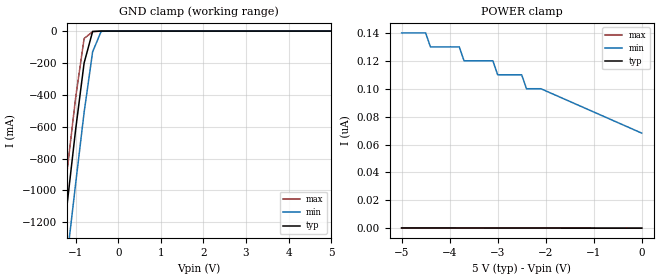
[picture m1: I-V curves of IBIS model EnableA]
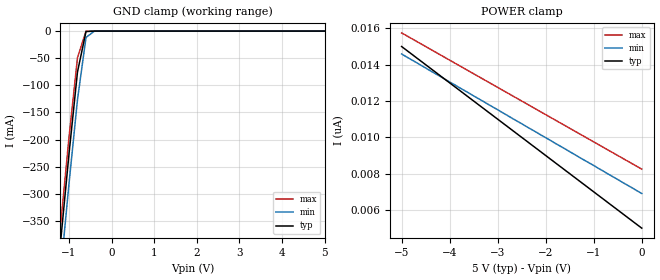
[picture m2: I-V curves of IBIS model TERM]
| I/O Buffer Information Specification (IBIS) Version 3.2 (August 20, 1999)
| IBIS is a standard for electronic behavioral specifications of integrated
| circuit input/output analog characteristics.
[IBIS Ver]   3.2
[File name]   qs3244.ibs
[File Rev]   2.0
[Date]   December 5, 2003
[Source]   From QSI silicon model
[Notes]   1. Temperatures: typ=25C, min=-40C, max=100C
   2. QSI's 0.8um SPDM process
   3. I/O model type changed to Series_switch for Data I/Os
[Disclaimer]
Integrated Device Technology, Inc. ("IDT") hereby grants the user of this
IBIS model ("User") a non-exclusive, nontransferable license to use this
IBIS model under the following terms: The User is granted this license only
to use the IBIS model for demonstration purposes only and is not granted
rights to sell, copy (except as needed to run the IBIS model), rent, lease
or sub-license (except for demonstration) the IBIS model in whole or in
part, or in modified form to anyone. The User may modify the IBIS model to
suit its specific applications, but  rights to derivative works and such
modifications shall belong to IDT.
THIS IBIS MODEL IS PROVIDED ON AN AS IS" BASIS AND IDT  MAKES ABSOLUTELY NO
WARRANTY WITH RESPECT TO THE INFORMATION CONTAINED HEREIN.  IDT DISCLAIMS
AND USER WAIVES ALL WARRANTIES, EXPRESS AND IMPLIED, INCLUDING WARRANTIES OF
MERCHANTABILITY AND FITNESS FOR A PARTICULAR PURPOSE.  THE ENTIRE RISK AS TO
QUALITY AND PERFORMANCE IS WITH THE USER  ACCORDINGLY, IN NO EVENT SHALL IDT
BE LIABLE FOR ANY DIRECT OR INDIRECT DAMAGES, WHETHER IN CONTRACT OR TORT,
INCLUDING ANY LOST PROFITS OR OTHER INCIDENTAL, CONSEQUENTIAL, EXEMPLARY, OR
PUNITIVE DAMAGES ARISING OUT OF THE USE OR APPLICATION OF THE  IBIS MODEL,
WHETHER OR NOT IDT HAD NOTICE OF SUCH DAMAGES.
IDT reserves the right to make changes without notice to any product herein
to improve reliability, function, or design. IDT does not convey any license
under patent rights or any other intellectual property rights, including
those of third parties. IDT is not obligated to provide maintenance or
support for the licensed IBIS model.
This model is for High Speed CMOS Quickswitch 8-Bit Bus Switch
[Copyright]
Copyright 2002, Integrated Device Technology, Inc. All rights reserved.
|   Component qs3244
[Component]   qs3244
[Manufacturer]   Quality Semiconductor Incorporated
[Package]
| Note that R_pkg is not given
| variable   typ   min   max
| Package parasitics.  Uncomment one set.
| PDIP
R_pkg   0.00   0.00   0.00
L_pkg   8.00nH   NA   NA
C_pkg   1.20pF   NA   NA
| SOIC
|R_pkg   0.00   0.00   0.00
|L_pkg   4.00nH   NA   NA
|C_pkg   0.70pF   NA   NA
| QSOP
|R_pkg   0.00   0.00   0.00
|L_pkg   2.50nH   NA   NA
|C_pkg   0.40pF   NA   NA
[Pin]  signal_name   model_name   R_pin   L_pin   C_pin
|1   ~1G   EnableA
2   1A1   TERM
3   2Y4   TERM
4   1A2   TERM
5   2Y3   TERM
6   1A3   TERM
7   2Y2   TERM
8   1A4   TERM
9   2Y1   TERM
11   2A1   TERM
12   1Y4   TERM
13   2A2   TERM
14   1Y3   TERM
15   2A3   TERM
16   1Y2   TERM
17   2A4   TERM
18   1Y1   TERM
|19   ~2G   EnableA
10   GND   GND
20   Vcc   POWER
[Series Switch Groups]
|Function Group States
On A /
On B /
On A B /
Off A B /
[Series Pin Mapping]   pin_2   model_name   function_table_group
2   18   QSW   A
4   16   QSW   A
6   14   QSW   A
8   12   QSW   A
11   9   QSW   B
13   7   QSW   B
15   5   QSW   B
17   3   QSW   B
|   Model QSW
[Model]   QSW
Model_type   Series_switch
C_comp   5.0pF   5.0pF   5.0pF
[Temperature Range]   25.00   100.00   -40.00
[Voltage Range]   5.00V   4.75V   5.25V
[On]
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[Off]
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| Models and submodels in the file (3): EnableA (Input), TERM (Terminator), QSW (Series_switch)
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|   Model EnableA
[Model]   EnableA
Model_type   Input
Vinl =   0.80V
Vinh =   2.00V
C_comp   5.00pF   5.00pF   5.00pF
[Temperature Range]   25.00   0.12k   -40.00
[Voltage Range]   5.00V   4.50V   5.50V
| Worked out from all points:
|   GND clamp passes 1 mA (typ) near -0.49 V on its own axis
[GND_clamp]
| voltage   I(typ)   I(min)   I(max)
-5V       -10.46A    -10.75A    -10.37A
-1.4V     -1.56A     -1.9A      -1.36A
-1.2V     -1.09A     -1.42A     -880mA
-1V       -620mA     -960mA     -420mA
-800mV    -200mA     -510mA     -46.44mA
-600mV    -2.14mA    -130mA     -4.03mA
-400mV    -3.69uA    -1.72mA    -40.62uA
5V        120pA      75.77nA    120pA
[POWER_clamp]
| voltage   I(typ)   I(min)   I(max)
-5V       280pA      140nA      290pA
-4.5V     270pA      140nA      280pA
-4.4V     260pA      130nA      270pA
-3.8V     240pA      130nA      250pA
-3.7V     240pA      120nA      250pA
-3.1V     220pA      120nA      230pA
-3V       220pA      110nA      230pA
-2.5V     200pA      110nA      210pA
-2.4V     200pA      100nA      210pA
-2.1V     190pA      100nA      200pA
0V        120pA      68.19nA    130pA
|   Model TERM
[Model]   TERM
Model_type   Terminator
Polarity   Non-Inverting
C_comp   5.00pF   5.00pF   5.00pF
[Temperature Range]   25.00   100.00   -40.00
[Voltage Range]   5.0V   4.75V   5.25V
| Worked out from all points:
|   GND clamp passes 1 mA (typ) near -0.60 V on its own axis
[GND_clamp]
| voltage   I(typ)   I(min)   I(max)M
-5V       -3.69A     -3.75A     -3.67A
-1.4V     -559.6mA   -614.8mA   -529.3mA
-1.2V     -391.1mA   -446.6mA   -360.7mA
-1V       -226.9mA   -282mA     -196.7mA
-800mV    -75.3mA    -126.3mA   -49.13mA
-600mV    -834.8uA   -11.75mA   -104.4uA
-400mV    -361.2nA   -21.26uA   -22.01nA
5V        10nA       7.68nA     7.5nA
[POWER_clamp]
| voltage   I(typ)   I(min)   I(max)
-5V       15nA       14.59nA    15.75nA
-4.4V     13.8nA     13.66nA    14.85nA
-3V       11nA       11.52nA    12.75nA
0V        5nA        6.91nA     8.25nA
